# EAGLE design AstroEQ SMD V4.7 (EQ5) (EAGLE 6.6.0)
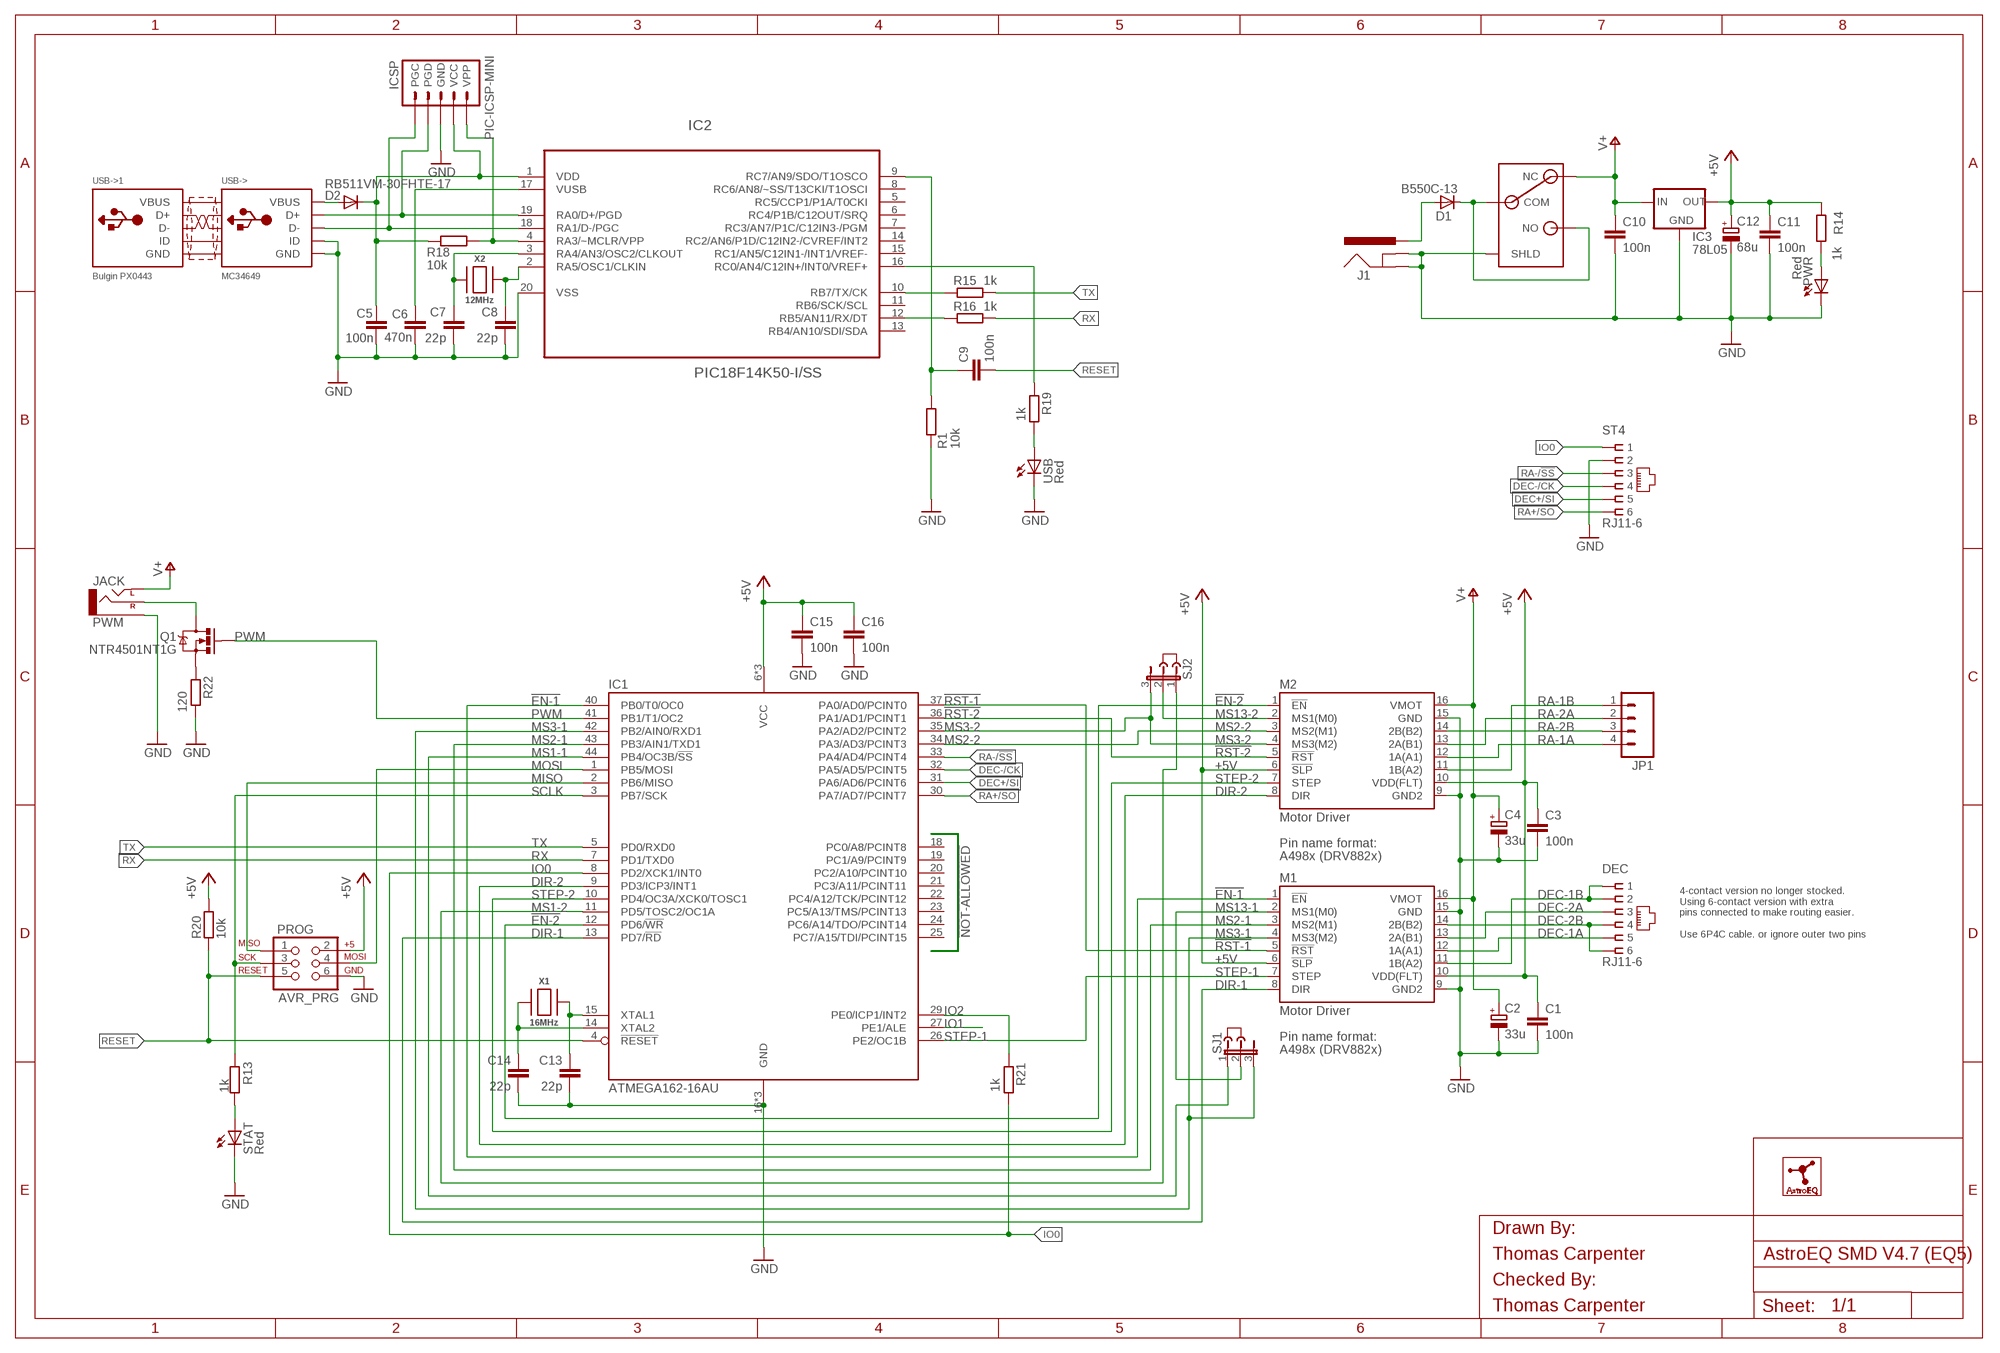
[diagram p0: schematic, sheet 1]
FRAME1 (A3L-LOC): CHECKED_BY: Thomas Carpenter; DRAWN_BY: Thomas Carpenter
USB->1 (USB-PANEL): MF: BULGIN; MPN: PX0443; OC_FARNELL: 1229685

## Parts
C1  100n  C-EUC0603  [C0603]
C2  33u  CPOL-EUSMCC  [SMC_C]
C3  100n  C-EUC0603  [C0603]
C4  33u  CPOL-EUSMCC  [SMC_C]
C5  100n  C-EUC0603  [C0603]
C6  470n  C-EUC0603  [C0603]
C7  22p  C-EUC0603  [C0603]
C8  22p  C-EUC0603  [C0603]
C9  100n  C-EUC0603  [C0603]
C10  100n  C-EUC0603  [C0603]
C11  100n  C-EUC0603  [C0603]
C12  68u  CPOL-EUSMCC  [SMC_C]
C13  22p  C-EUC0603  [C0603]
C14  22p  C-EUC0603  [C0603]
C15  100n  C-EUC0603  [C0603]
C16  100n  C-EUC0603  [C0603]
D1  B550C-13  DIODE-SMC  [SMC]
D2  RB511VM-30FHTE-17  DIODESOD  [SOD-323]
DEC  RJ11-6  RJ11-2L-B  [RJ11-NO_SHIELD]
IC1  ATMEGA162-16AU  [TQFP44]
IC2  PIC18F14K50-I/SS  [SS20]
IC3  78L05  78LXXSOT-23  [SOT23]
ICSP  PIC-ICSP-MINI  [PIC-ICSP-MINI]
J1  POWER_JACKPANEL  [POWER_JACK_PANEL]
J2  JUMPER  [JUMP]
J3  JUMPER  [JUMP]
JP1  M04POLAR  [MOLEX-1X4]
LOGO1  ASTROEQ5MM  [ASTROEQ-SMALL]
M1  Motor Driver  A4983CARRIER  [DIP16-W]
M2  Motor Driver  A4983CARRIER  [DIP16-W]
PROG  AVR_PRG  AVR_SPI_PRG_6PTH  [2X3]
PWM  JACK  AUDIO-JACKVERT  [AUDIO-JACK-3.5MM-VERT]
PWR  Red  LED3MM  [LED3MM]
PWR-SW  SWITCH  [SPST]
Q1  NTR4501NT1G  MOSFET-NCHANNELSMD  [SOT23-3]
R1  10k  R-EU_R0603  [R0603]
R13  1k  R-EU_R0603  [R0603]
R14  1k  R-EU_R0603  [R0603]
R15  1k  R-EU_R0603  [R0603]
R16  1k  R-EU_R0603  [R0603]
R18  10k  R-EU_R0603  [R0603]
R19  1k  R-EU_R0603  [R0603]
R20  10k  R-EU_R0603  [R0603]
R21  1k  R-EU_R0603  [R0603]
R22  120  R-EU_R0805  [R0805]
SJ1  JP2E  [JP2]
SJ2  JP2E  [JP2]
ST4  RJ11-6  RJ11-2L-B  [RJ11-NO_SHIELD]
STAT  Red  LED3MM  [LED3MM]
USB  Red  LED3MM  [LED3MM]
USB->  MC34649  USBBULGINWIRE  [22-23-2051]
X1  16MHz  XTALNX5032  [NX5032]
X2  12MHz  XTALNX5032  [NX5032]

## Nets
!EN-1: IC1.40(PB0/T0/OC0) M1.1(!EN)
!EN-2: IC1.12(PD6/!WR) M2.1(!EN)
!RST-1: IC1.37(PA0/AD0/PCINT0) M1.5(!RST)
!RST-2: IC1.36(PA1/AD1/PCINT1) M2.5(!RST)
+5V: C1.1 C3.1 C11.1 C12.+ C15.1 C16.1 IC1.6(VCC) IC1.17(VCC) IC1.38(VCC) IC3.1(OUT) M1.6(!SLP) M1.10(VDD(FLT)) M2.6(!SLP) M2.10(VDD(FLT)) PROG.2 R14.1 R20.2
AVROSC1: C13.1 IC1.15(XTAL1) X1.P$1
AVROSC2: C14.1 IC1.14(XTAL2) X1.P$2
D_N [usbdat]: IC2.18(RA1/D-/PGC) ICSP.5(PGC) USB->.2(D-)
D_P [usbdat]: IC2.19(RA0/D+/PGD) ICSP.4(PGD) USB->.3(D+)
DEC+/SI: IC1.31(PA6/AD6/PCINT6) ST4.5
DEC-1A: DEC.5 M1.12(1A(A1))
DEC-1B: DEC.1 DEC.2 M1.11(1B(A2))
DEC-2A: DEC.3 M1.13(2A(B1))
DEC-2B: DEC.4 DEC.6 M1.14(2B(B2))
DEC-/CK: IC1.32(PA5/AD5/PCINT5) ST4.4
DIR-1: IC1.13(PD7/!RD) M1.8(DIR)
DIR-2: IC1.9(PD3/ICP3/INT1) M2.8(DIR)
DTR: C9.1 IC2.9(RC7/AN9/SDO/T1OSCO) R1.1
GND: C1.2 C2.- C3.2 C4.- C5.2 C6.1 C7.2 C8.2 C10.2 C11.2 C12.- C13.2 C14.2 C15.2 C16.2 IC1.16(GND) IC1.28(GND) IC1.39(GND) IC2.20(VSS) IC3.3(GND) ICSP.3(GND) J1.SHUNT(GNDBREAK) J1.SLEEVE(GND) M1.9(GND2) M1.15(GND) M2.9(GND2) M2.15(GND) PROG.6 PWM.1(SLEEVE) PWR-SW.S1(SHLD) PWR-SW.S2(SHLD) PWR-SW.S3(SHLD) PWR-SW.S4(SHLD) PWR.K(C) R1.2 R22.1 ST4.2 STAT.K(C) USB->.4(GND) USB->.5(ID) USB.K(C)
IO0: IC1.8(PD2/XCK1/INT0) R21.1 ST4.1
IO1: IC1.27(PE1/ALE)
IO2: IC1.29(PE0/ICP1/INT2) R21.2
MCLR: IC2.4(RA3/~MCLR/VPP) ICSP.1(VPP) R18.1
MISO: IC1.2(PB6/MISO) PROG.1
MOSI: IC1.1(PB5/MOSI) PROG.4
MS1-1: IC1.44(PB4/OC3B/!SS) SJ1.1
MS1-2: IC1.11(PD5/TOSC2/OC1A) SJ2.1
MS2-1: IC1.43(PB3/AIN1/TXD1) M1.3(MS2(M1))
MS2-2: IC1.34(PA3/AD3/PCINT3) M2.3(MS2(M1))
MS3-1: IC1.42(PB2/AIN0/RXD1) M1.4(MS3(M2)) SJ1.3
MS3-2: IC1.35(PA2/AD2/PCINT2) M2.4(MS3(M2)) SJ2.3
MS13-1: M1.2(MS1(M0)) SJ1.2
MS13-2: M2.2(MS1(M0)) SJ2.2
PWM: IC1.41(PB1/T1/OC2) Q1.1(G)
PWM-OUT: PWM.3(RIGHT) Q1.3(D)
PWM-RES: Q1.2(S) R22.2
PWRLED: PWR.A R14.2
RA+/SO: IC1.30(PA7/AD7/PCINT7) ST4.6
RA-1A: JP1.4 M2.12(1A(A1))
RA-1B: JP1.1 M2.11(1B(A2))
RA-2A: JP1.2 M2.13(2A(B1))
RA-2B: JP1.3 M2.14(2B(B2))
RA-/!SS: IC1.33(PA4/AD4/PCINT4) ST4.3
RESET: C9.2 IC1.4(!RESET) PROG.5 R20.1
RX: IC1.7(PD1/TXD0) R16.1
RX(USB): IC2.12(RB5/AN11/RX/DT) R16.2
SCLK: IC1.3(PB7/SCK) PROG.3 R13.1
STATLED: R13.2 STAT.A
STEP-1: IC1.26(PE2/OC1B) M1.7(STEP)
STEP-2: IC1.10(PD4/OC3A/XCK0/TOSC1) M2.7(STEP)
SWITCH: D1.C PWR-SW.COM PWR-SW.NO
TX: IC1.5(PD0/RXD0) R15.1
TX(USB): IC2.10(RB7/TX/CK) R15.2
USBLED: R19.1 USB.A
USBOSC1: C8.1 IC2.2(RA5/OSC1/CLKIN) X2.P$2
USBOSC2: C7.1 IC2.3(RA4/AN3/OSC2/CLKOUT) X2.P$1
USBSTAT: IC2.16(RC0/AN4/C12IN+/INT0/VREF+) R19.2
V+: C2.+ C4.+ C10.1 IC3.2(IN) M1.16(VMOT) M2.16(VMOT) PWM.2(LEFT) PWR-SW.NC
VBUS: D2.2(A) USB->.1(VBUS)
VIN: D1.A J1.CENTRE(PWR)
VPIC: C5.1 D2.1(C) IC2.1(VDD) ICSP.2(VCC) R18.2
VUSB: C6.2 IC2.17(VUSB)
Unconnected: IC1.18(PC0/A8/PCINT8) IC1.19(PC1/A9/PCINT9) IC1.20(PC2/A10/PCINT10) IC1.21(PC3/A11/PCINT11) IC1.22(PC4/A12/TCK/PCINT12) IC1.23(PC5/A13/TMS/PCINT13) IC1.24(PC6/A14/TDO/PCINT14) IC1.25(PC7/A15/TDI/PCINT15) IC2.5(RC5/CCP1/P1A/T0CKI) IC2.6(RC4/P1B/C12OUT/SRQ) IC2.7(RC3/AN7/P1C/C12IN3-/PGM) IC2.8(RC6/AN8/~SS/T13CKI/T1OSCI) IC2.11(RB6/SCK/SCL) IC2.13(RB4/AN10/SDI/SDA) IC2.14(RC2/AN6/P1D/C12IN2-/CVREF/INT2) IC2.15(RC1/AN5/C12IN1-/INT1/VREF-)

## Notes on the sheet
- 4-contact version no longer stocked.
  Using 6-contact version with extra
  pins connected to make routing easier.
  
  Use 6P4C cable. or ignore outer two pins

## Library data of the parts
C1 C3 C5 C9-C11 C15 C16 = rcl:C-EU: CAPACITOR, European symbol; MF: MULTICOMP; MPN: MC0603F104Z250CT; OC_FARNELL: 1759038
C2 C4 = rcl:CPOL-EU: POLARIZED CAPACITOR, European symbol; MF: KEMET; MPN: T491C336K025AT; OC_FARNELL: 1793896
C6 = rcl:C-EU: CAPACITOR, European symbol; MF: MULTICOMP; MPN: MC0603F474Z160CT; OC_FARNELL: 1759021
C7 C8 C13 C14 = rcl:C-EU: CAPACITOR, European symbol; MF: MULTICOMP; MPN: MC0603N220J500CT; OC_FARNELL: 1759057
C12 = rcl:CPOL-EU: POLARIZED CAPACITOR, European symbol; MF: AVX; MPN: TPSC686K016R0125; OC_FARNELL: 1658976
D1 = diode:DIODE-: DIODE; MF: DIODES INC.; MPN: B550C-13-F; OC_FARNELL: 1858608
D2 = SparkFun:DIODE: Diode; MF: ROHM; MPN: RB511VM-30FHTE-17; OC_FARNELL: 2581544
DEC ST4 = con-tycoelectronics:RJ11: CORCOM Modular RJ Jacks No Shield Source: www.tycoelectronics.com .. ENG_DS_1654001_1099_RJ_L_0507.pdf; MF: MOLEX; MPN: 95503-2661; OC_FARNELL: 1620210
IC1 = atmel:ATMEGA162: 8-bit RISC MICROCONTROLLER 16K Bytes internal flash program memory 1K Bytes internal SRAM Upto 64K Bytes optional external memory space 512 Bytes EEPROM Two 8-bit timers Two 16-bit timers Dual programmable serial USARTs Master/Slave serial SPI interface Source: ATMEGA162_DIP40.lbr; MF: ATMEL; MPN: ATMEGA162-16AU; OC_FARNELL: 9171150
IC2 = microchip:PIC18F14K50: USB Flash Microcontrollers; MF: MICROCHIP
IC3 = v-reg:78LXX: VOLTAGE REGULATOR; MF: TAIWAN SEMICONDUCTOR; MPN: TS78L05CX RFG; OC_FARNELL: 1476698
ICSP = SparkFun:PIC-ICSP-MINI: PIC-ICSP-Mini Miniature 5-pin connection for temporary programming of PICs. Use this device in your design to save space. Program the PIC with this adapter Spark Fun Electronics SKU : BOB-00194; OC_FARNELL: unknown
J1 = SparkFun:POWER_JACK: Power Jack This is the standard 5.5mm barrel jack for power. The PTH is the most common, proven, reliable, footprint. All others are experimental. The Slot footprint only works if the mill layer is transmitted to the PCB fab house so be warned. Spark Fun Electronics SKU : PRT-00119. Mating wall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; MF: SWITCHCRAFT; MPN: PCL712AS; OC_FARNELL: 1871167
J2 J3 = jumper:JUMPER: JUMPER header; MF: 3M; MPN: 969102-0000-DA; OC_FARNELL: 2579814
JP1 = SparkFun:M04: Header 4 Standard 4-pin 0.1" header. Use with straight break away headers (SKU : PRT-00116), right angle break away headers (PRT-00553), swiss pins (PRT-00743), machine pins (PRT-00117), and female headers (PRT-00115). Molex polarized connector foot print use with SKU : PRT-08231 with associated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; MF: MULTICOMP; MPN: MC34645; OC_FARNELL: 1675775
LOGO1 = AstroEQTooth:ASTROEQ; OC_FARNELL: unknown
M1 M2 = A4983Carrier:A4983CARRIER; MF: SAMTEC; MPN: CES-116-01-T-S; OC_FARNELL: 1667522
PROG = SparkFun:AVR_SPI_PRG_6: AVR ISP 6 Pin This is the reduced ISP connector for AVR programming. Common on Arduino. This footprint will take up less PCB space and can be used with a 10-pin to 6-pin adapter such as SKU: BOB-08508; MF: AMP - TE CONNECTIVITY; MPN: 826632-3; OC_FARNELL: 3418492
PWM = SparkFun:AUDIO-JACK: 3.5mm Audio Jack Simple 3.5mm common PCB mount audio jack. SKU: PRT-08032; MANUFACTURER: LUMBERG; MF: LUMBERG; MPN: 1502 01; OC_FARNELL: 1243242
PWR STAT USB = led:LED: LED; MF: KINGBRIGHT; MPN: L-424HDT; OC_FARNELL: 1142499
PWR-SW = con-tycoelectronics:SWITCH; MF: TE CONNECTIVITY; MPN: AE101J1V3B004; OC_FARNELL: 1813654
Q1 = SparkFun:MOSFET-NCHANNEL; MF: ON SEMICONDUCTOR; MPN: NTR4501NT1G; OC_FARNELL: 1431305
R1 R18 R20 = rcl:R-EU_: RESISTOR, European symbol; MF: MULTICOMP; MPN: MCWR06X1002FTL; OC_FARNELL: 2447230
R13-R16 R19 R21 = rcl:R-EU_: RESISTOR, European symbol; MF: MULTICOMP; MPN: MCWR06X1001FTL; OC_FARNELL: 2447272
R22 = rcl:R-EU_: RESISTOR, European symbol; MF: MULTICOMP; MPN: MCWR08X1200FTL; OC_FARNELL: 2447561
SJ1 SJ2 = jumper:JP2E: JUMPER; MF: MULTICOMP; MPN: 2211S-03G; OC_FARNELL: 1593412
USB-> = adafruit:USB: USB Connectors USBMINIB - Surface Mount Female Mini-B USB Connector 4UConnector: 06564 By microbuilder.eu Thru-hole RA Female Mini-B USB Connector 4UConnector: 18732 By ladyada.net; MF: MULTICOMP; MPN: MC34649; OC_FARNELL: 1675777
X1 = adafruit:XTAL: Low cost SMT crystals, no capacitors included; MF: TXC; MPN: 7A-16.000MAAJ-T; OC_FARNELL: 1841946
X2 = adafruit:XTAL: Low cost SMT crystals, no capacitors included; MF: TXC; MPN: 7A-12.000MAAJ-T; OC_FARNELL: 1841940

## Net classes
1 power: width 0.61 mm, drill 0.711 mm, clearance 0.203 mm
2 gnd: width 0.305 mm, drill 0.711 mm, clearance 0.203 mm
3 usbvcc: width 0.508 mm, drill 0.711 mm, clearance 0.203 mm
4 usbdat: width 0.406 mm, clearance 0.152 mm

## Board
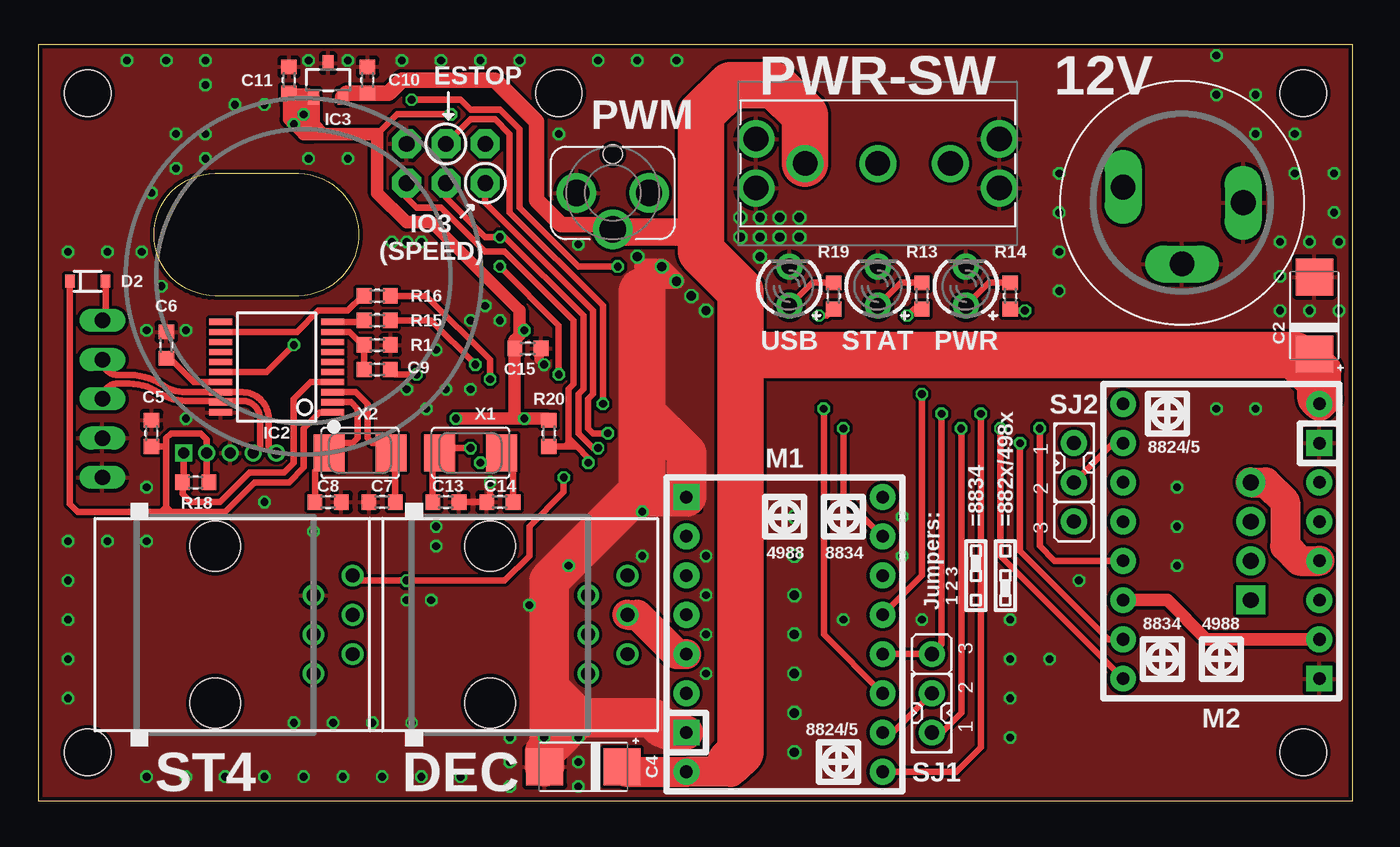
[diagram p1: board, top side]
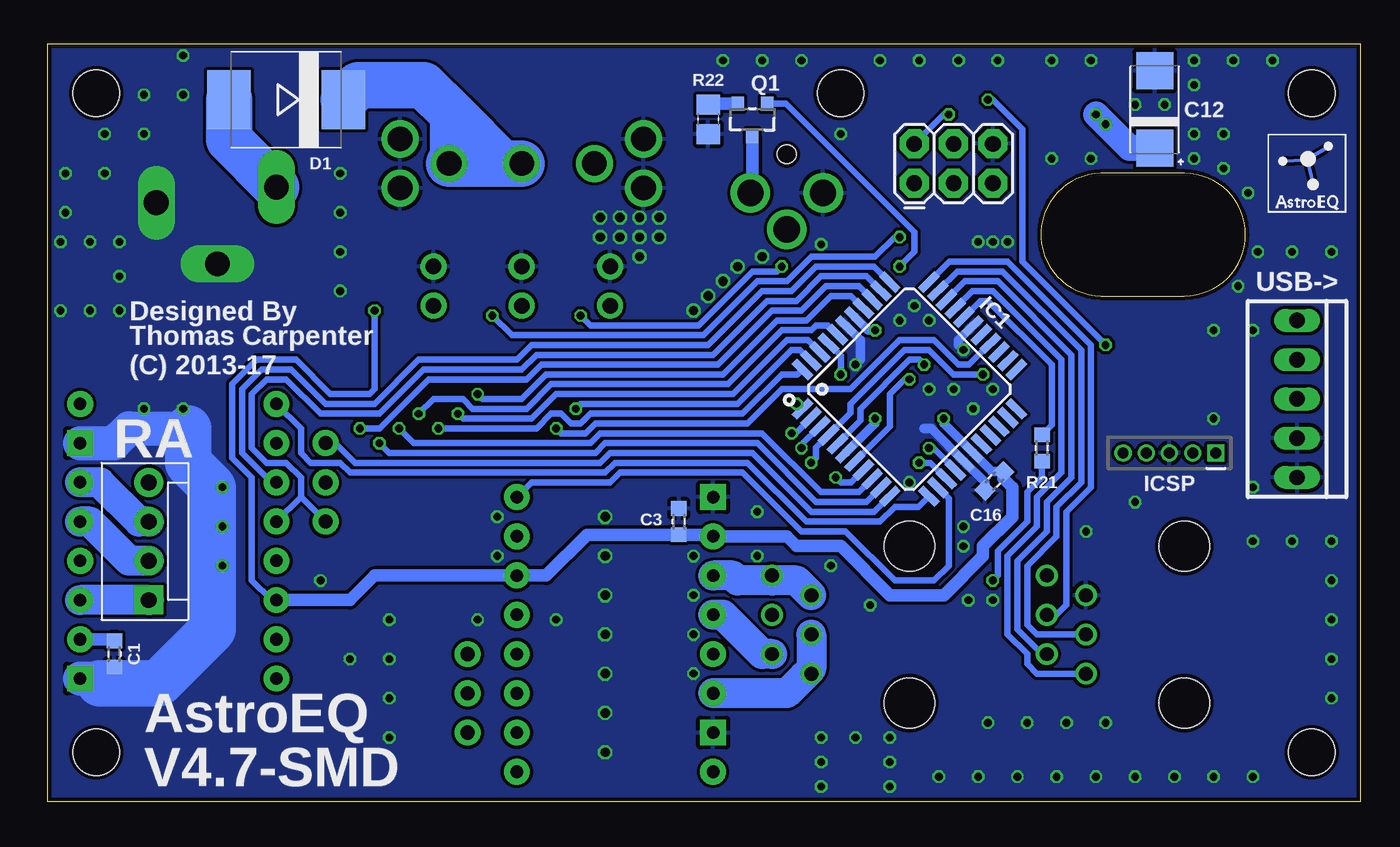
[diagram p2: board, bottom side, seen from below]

Size 85 x 49 mm. Coordinates in mm from the lower left corner, seen from the top.
Outline: 0,0 0,49 85,49 85,0 0,0
Outline: 16.83,40.64 arc-177 16.83,32.7 11.43,32.7 arc-180 11.43,40.64 16.83,40.64
Copper layers (1*16): Top 0.035mm / dielectric 1.5mm / Bottom 0.035mm
Design rules "ITEADstudio_DRC *": minimum track width 6mil, minimum drill 12mil, track to track 6mil, track to pad 6mil, pad to pad 6mil, via to via 6mil, smd to smd 0mil, copper to edge 10mil, drill to drill 10mil, minimum pad ring 8mil, minimum via ring 6mil, stop-mask expansion 2mil, vias tented up to drill 1mm, thermal gap 10mil
Holes 3 mm at 81.83,3.17 33.66,45.83 3.17,45.83 81.83,45.83 3.17,3.17

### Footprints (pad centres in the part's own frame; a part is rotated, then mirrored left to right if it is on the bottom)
C0603 = smd 0.95 x 1: 1 -0.85,0; 2 0.85,0
SMC_C = smd 2.4 x 2.4: + -2.5,0; - 2.5,0
SMC = smd 2.8 x 3.8: A 3.7,0; C -3.7,0
SOD-323 = smd 0.63 x 0.83: 1 -1.15,0; 2 1.15,0
RJ11-NO_SHIELD = drill 0.9 pad 1.4: 1 -3.175,8.89; 2 -1.905,6.35; 3 -0.635,8.89; 4 0.635,6.35; 5 1.905,8.89; 6 3.175,6.35 | hole 3.251: -5.08,0; 5.08,0
TQFP44 = smd 1.5 x 0.5: 1 -5.8,4; 2 -5.8,3.2; 3 -5.8,2.4; 4 -5.8,1.6; 5 -5.8,0.8; 6 -5.8,0; 7 -5.8,-0.8; 8 -5.8,-1.6; 9 -5.8,-2.4; 10 -5.8,-3.2; 11 -5.8,-4; 23 5.8,-4; 24 5.8,-3.2; 25 5.8,-2.4; 26 5.8,-1.6; 27 5.8,-0.8; 28 5.8,0; 29 5.8,0.8; 30 5.8,1.6; 31 5.8,2.4; 32 5.8,3.2; 33 5.8,4 | smd 0.5 x 1.5: 12 -4,-5.8; 13 -3.2,-5.8; 14 -2.4,-5.8; 15 -1.6,-5.8; 16 -0.8,-5.8; 17 0,-5.8; 18 0.8,-5.8; 19 1.6,-5.8; 20 2.4,-5.8; 21 3.2,-5.8; 22 4,-5.8; 34 4,5.8; 35 3.2,5.8; 36 2.4,5.8; 37 1.6,5.8; 38 0.8,5.8; 39 0,5.8; 40 -0.8,5.8; 41 -1.6,5.8; 42 -2.4,5.8; 43 -3.2,5.8; 44 -4,5.8
SS20 = smd 0.4 x 1.5: 1 -2.925,-3.625; 2 -2.275,-3.625; 3 -1.625,-3.625; 4 -0.975,-3.625; 5 -0.325,-3.625; 6 0.325,-3.625; 7 0.975,-3.625; 8 1.625,-3.625; 9 2.275,-3.625; 10 2.925,-3.625; 11 2.925,3.625; 12 2.275,3.625; 13 1.625,3.625; 14 0.975,3.625; 15 0.325,3.625; 16 -0.325,3.625; 17 -0.975,3.625; 18 -1.625,3.625; 19 -2.275,3.625; 20 -2.925,3.625
SOT23 = smd 0.7 x 1: 1 -0.95,-1.1; 2 0.95,-1.1; 3 0,1.1
PIC-ICSP-MINI = drill 0.7 square: 1 -3,0 | drill 0.7: 2 -1.5,0; 3 0,0; 4 1.5,0; 5 3,0
POWER_JACK_PANEL = drill 1.6 long: CENTRE 3.81,-1.016; SHUNT -3.962,0; SLEEVE 0,3.962
MOLEX-1X4 = drill 1.016 pad 1.88 square: 1 0,0 | drill 1.016 pad 1.88: 2 2.54,0; 3 5.08,0; 4 7.62,0
DIP16-W = drill 0.813 pad 1.676: 1 -8.89,-6.35; 2 -6.35,-6.35; 3 -3.81,-6.35; 4 -1.27,-6.35; 5 1.27,-6.35; 6 3.81,-6.35; 7 6.35,-6.35; 8 8.89,-6.35; 10 6.35,6.35; 11 3.81,6.35; 12 1.27,6.35; 13 -1.27,6.35; 14 -3.81,6.35; 16 -8.89,6.35 | drill 0.813 pad 1.676 square: 9 8.89,6.35; 15 -6.35,6.35
2X3 = drill 1.016 pad 1.88 octagon: 1 -2.54,-1.27; 2 -2.54,1.27; 3 0,-1.27; 4 0,1.27; 5 2.54,-1.27; 6 2.54,1.27
AUDIO-JACK-3.5MM-VERT = drill 1.7: 1 2.35,0; 2 0,2.35; 3 -2.35,0 | hole 1.2: 0,-2.5
LED3MM = drill 1 pad 1.676: A -1.27,0; K 1.27,0
SPST = drill 1.6: COM 0,0; NC -4.699,0; NO 4.699,0; S1 7.874,1.587; S2 7.874,-1.587; S3 -7.874,1.587; S4 -7.874,-1.587
SOT23-3 = smd 0.8 x 0.9: 1 -0.95,-1; 2 0.95,-1; 3 0,1.1
R0603 = smd 0.95 x 1: 1 -0.85,0; 2 0.85,0
R0805 = smd 1.3 x 1.5: 1 -0.95,0; 2 0.95,0
JP2 = drill 0.914 pad 1.676: 1 -2.54,0; 2 0,0; 3 2.54,0
22-23-2051 = drill 1 long: 1 -5.08,0; 2 -2.54,0; 3 0,0; 4 2.54,0; 5 5.08,0
NX5032 = smd 2 x 2.4: P$1 2,0; P$2 -2,0

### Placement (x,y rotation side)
C1  80.64,9.53 270 bottom
C2  82.55,31.43 90 top
C3  44.13,18.1 90 bottom
C4  35.24,2.22 180 top
C5  7.3,23.81 90 top
C6  8.26,29.53 270 top
C7  22.23,19.37 180 top
C8  18.73,19.37 0 top
C9  21.91,27.94 0 top
C10  21.27,46.67 90 top
C11  16.19,46.67 90 top
C12  13.34,44.77 90 bottom
C13  26.35,19.37 0 top
C14  29.84,19.37 180 top
C15  31.66,29.3 0 top
C16  23.72,20.73 225 bottom
D1  69.53,45.4 180 bottom
D2  3.17,33.66 0 top
DEC  29.21,11.43 270 top
IC1  29.21,26.67 45 bottom
IC2  15.4,28.1 90 top
IC3  18.73,46.67 0 top
ICSP  12.38,22.54 180 bottom
J1  73.98,38.73 180 top
J2  57.78,5.71 0 top
J3  66.99,21.91 0 top
JP1  78.42,13.02 90 bottom
LOGO1  6.03,38.1 0 bottom
M1  48.26,10.79 90 top
M2  76.52,16.83 270 top
PROG  26.35,41.27 0 bottom
PWM  37.15,39.37 180 top
PWR  60.01,33.34 90 top
PWR-SW  54.29,41.27 0 top
Q1  39.37,44.13 180 bottom
R1  21.91,29.53 0 top
R13  57.15,32.7 90 top
R14  62.87,32.7 90 top
R15  21.91,31.11 180 top
R16  21.91,32.7 180 top
R18  10.16,20.64 0 top
R19  51.44,32.7 270 top
R20  33.02,23.81 90 top
R21  20.64,22.86 90 bottom
R22  42.23,44.13 90 bottom
SJ1  57.78,6.99 90 top
SJ2  66.99,20.64 270 top
ST4  11.43,11.43 270 top
STAT  54.29,33.34 90 top
USB  48.58,33.34 90 top
USB->  4.13,26.04 270 bottom
X1  27.94,22.54 180 top
X2  20.8,22.54 0 top

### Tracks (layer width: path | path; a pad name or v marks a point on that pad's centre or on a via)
!EN-1  (via drill 0.5)
  Top 0.406: M1.1 59.37,1.91 60.96,3.49 v60.96,25.08
  Bottom 0.406: IC1.40 34.47,30.8 35.24,30.8 35.56,30.48 37.47,30.48 40.96,26.99 52.39,26.99 53.98,25.4 57.47,25.4 58.1,26.04 60.01,26.04 v60.96,25.08
!EN-2
  Bottom 0.406: IC1.12 28.63,19.05 30.16,19.05 31.11,18.1 35.88,18.1 39.69,21.91 48.26,21.91 48.9,21.27 65.41,21.27 66.04,21.91 67.94,21.91 68.58,22.54 68.58,24.13 M2.1
!RST-1  (via drill 0.5)
  Top 0.406: M1.5 57.15,14.61 v57.15,26.35
  Bottom 0.406: IC1.37 32.98,32.7 34.29,32.7 35.88,31.11 37.78,31.11 41.27,27.62 52.7,27.62 54.29,26.04 56.83,26.04 v57.15,26.35
!RST-2  (via drill 0.5)
  Top 0.406: M2.5 65.72,15.56 64.77,16.51 v64.77,24.13
  Bottom 0.406: IC1.36 32.48,33.34 34.61,33.34 36.2,31.75 38.1,31.75 41.59,28.26 53.02,28.26 53.98,27.3 60.33,27.3 63.5,24.13 v64.77,24.13
+5V  (via drill 0.5)
  Top 0.406: 31.11,30.16 30.8,29.84 | v26.67,44.45 23.18,44.45 21.91,43.18 | R14.1 62.97,31.75 v63.82,31.75
  Top 0.813: R20.2 32.92,24.77 v31.43,24.77 30.8,24.77 | v26.99,24.77 30.8,24.77 | 30.8,24.77 30.8,29.29 C15.1 30.81,29.86 v31.43,30.48 31.11,30.8 | 31.11,30.8 31.11,31.75 25.4,37.47 23.81,37.47 21.91,39.37 21.91,43.18 18.41,43.18 | 31.11,30.8 31.11,30.16 | M2.6 73.03,13.02 75.56,10.48 M2.10 | 18.41,43.18 17.78,43.81 | 17.78,43.81 IC3.1 | 16.19,45.4 C11.1 16.41,45.82 16.51,45.72 | 16.19,45.4 16.83,44.77 16.83,44.45 16.19,45.09 | 16.19,45.09 16.19,45.4 | 16.19,45.09 16.19,44.13 v16.51,43.81 17.14,43.18 17.78,43.18 | 18.41,43.18 17.78,43.18 | 17.78,43.18 17.14,43.81 v17.14,44.45 17.78,43.81 | 16.51,45.72 17.78,44.45 17.78,45.4 17.46,45.72 16.51,45.72
  Bottom 0.406: PROG.2 26.99,44.45 v26.67,44.45 | v63.82,31.75 63.82,26.67 64.14,26.35 66.67,26.35 68.9,28.57 71.44,28.57 73.03,26.99 73.03,22.23 71.75,20.95 71.75,14.29 70.48,13.02 M2.6
  Bottom 0.61: C16.1 23.87,21.33 IC1.17 26.99,24.45 v26.99,24.77 | v31.43,24.77 31.43,24.45 IC1.6 | IC1.38 31.89,30.48 v31.43,30.48
  Bottom 0.813: C16.1 23.12,20.9 22.54,20.32 22.54,18.41 24.45,16.51 24.45,15.88 26.99,13.34 30.48,13.34 33.66,16.51 36.51,16.51 37.15,17.14 M1.10 42.01,17.25 C3.1 50.06,17.25 52.7,14.61 M1.6 63.82,14.61 65.41,13.02 M2.6 | 80.54,10.48 C1.1 80.75,10.48 M2.10
  Bottom 1.676: C12.+ 14.96,42.27 v17.14,44.45
AVROSC1  (via drill 0.5)
  Top 0.406: v27.94,22.86 26.26,22.86 X1.P$1 25.5,22.11 C13.1
  Bottom 0.406: IC1.15 27.66,22.86 v27.94,22.86
AVROSC2  (via drill 0.5)
  Top 0.406: v28.57,21.91 29.3,21.91 X1.P$2 30.7,21.79 C14.1
  Bottom 0.406: IC1.14 27.84,21.91 v28.57,21.91
D_N
  Top 0.406: USB->.2 arc90 5.12,27.58 5.87,27.58 arc-34 8.1,26.9 arc35 9.52,26.47 IC2.18 | ICSP.5 arc-90 14.88,23.04 14.88,24.77 arc90 13.18,26.47 IC2.18 | IC2.18
D_P
  Top 0.406: USB->.3 arc-90 5.12,27.03 5.87,27.03 arc-34 7.78,26.44 arc35 9.53,25.91 11.77,25.91 | ICSP.4 arc90 14.33,22.99 14.33,24.77 arc90 13.18,25.91 11.77,25.91 | IC2.19 11.77,25.91
DEC+/SI
  Bottom 0.406: IC1.31 25.62,33.66 23.5,33.66 18.73,28.89 18.73,20.95 20.32,19.37 20.32,17.46 22.23,15.56 22.23,11.11 20.64,9.53 ST4.5
DEC-1A
  Bottom 1.93: DEC.5 38.73,9.53 41.27,12.06 M1.12
DEC-1B
  Bottom 0.406: DEC.1 38.1,14.29
  Bottom 1.93: DEC.2 36.51,14.29 38.1,14.29 40.32,14.29 40.64,14.61 M1.11
DEC-2A
  Top 1.93: DEC.3 38.73,12.06 41.27,9.53 M1.13
DEC-2B
  Bottom 0.406: DEC.6 36.04,8.26 36.04,8.1
  Bottom 1.93: DEC.4 35.56,8.57 36.04,8.1 37.15,6.99 M1.14
DEC-/CK
  Bottom 0.406: IC1.32 26.11,34.29 23.18,34.29 18.1,29.21 18.1,20.64 19.68,19.05 19.68,17.14 21.59,15.24 21.59,11.43 20.95,10.79 ST4.4
DIR-1
  Bottom 0.406: IC1.13 26.67,19.61 26.67,15.24 27.62,14.29 30.16,14.29 33.34,17.46 36.2,17.46 40.01,21.27 47.94,21.27 48.58,20.64 53.66,20.64 M1.8
DIR-2  (via drill 0.5)
  Top 0.406: M2.8 62.23,15.88 v62.23,24.13
  Bottom 0.406: IC1.9 32.48,20 34.92,20 38.73,23.81 49.21,23.81 49.85,23.18 61.28,23.18 v62.23,24.13
DTR
  Top 0.406: IC2.9 20.11,30.37 20.95,29.53 R1.1 C9.1
GND  (via drill 0.5, 0.6)
  Top 0.406: C13.2 C14.2 29.21,19.58 v29.21,20.64
  Top 0.61: C15.2 32.38,29.18 32.38,28.57 v32.7,28.26
  Top 1.016: 39.05,34.61 v40.32,34.61 v41.27,33.66 38.42,33.66 38.42,33.02 39.05,33.02
  Top 2.184: 40.32,4.76 40.64,4.45 M1.15
  Top 2.54: C4.- 32.74,3.21 33.02,3.49 | 33.02,3.49 34.92,5.4 | 34.92,5.4 39.69,5.4 40.32,4.76 | 34.92,5.4 33.02,7.3 | 33.02,7.3 33.02,14.29 38.42,19.68 M1.9 41.91,22.54 39.05,25.4 | 33.02,7.3 33.02,3.49
  Top 3: 39.05,20.32 39.05,25.4 39.05,33.02
  Bottom 0.61: C16.2 24.32,20.65 IC1.16 27.8,24.13 28.26,24.13 | IC1.28 26.04,29.84 26.04,29.53 v25.72,29.21 | IC1.39 32.38,29.84 32.38,28.57 v32.7,28.26
  Bottom 0.813: C1.2 81.38,7.94
  Bottom 2.184: 81.38,7.94 M2.9 | M2.15 80.64,23.18 79.69,24.13 75.88,24.13
  Bottom 3: 75.88,24.13 75.88,21.91 74.3,20.32 74.3,11.11 77.79,7.62 81.6,7.62
  other vias: 14.61,19.37 17.78,17.46 25.72,17.78 9.53,24.77 9.53,30.48 25.72,16.51 47.94,36.51 43.18,31.75 46.67,35.24 23.81,26.67 27.94,26.67 27.94,31.11 29.84,31.11 25.08,25.4 26.35,26.67 45.4,36.51 46.67,36.51 22.86,36.2 28.89,32.07 49.21,36.51 47.94,37.78 49.21,37.78 45.4,37.78 46.67,37.78 42.23,32.7 48.9,3.17 48.9,5.71 48.9,8.26 48.9,10.79 48.9,13.34 48.9,15.88 48.9,18.41 23.81,13.02 25.4,13.02 34.29,15.24 39.05,18.73 30.48,0.95 30.48,4.13 34.92,4.13 34.92,0.95 32.7,4.13 30.48,2.54 34.92,2.54 43.18,8.26 43.18,10.79 43.18,13.34 43.18,15.88 39.05,15.88 38.73,35.24 23.81,36.2 24.77,36.2 34.92,36.04 84.14,36.2 84.14,31.75 82.23,36.2 80.33,36.2 80.33,33.97 80.33,31.75 82.23,31.75 10.79,47.94 10.79,46.35 12.7,45.09 14.61,45.09 17.46,47.94 20,47.94 23.5,47.94 26.04,47.94 28.57,47.94 31.11,47.94 36.2,47.94 38.73,47.94 41.27,47.94 33.66,43.18 7.94,33.34 8.89,40.96 8.89,43.18 10.79,43.18 20,41.59 1.91,16.83 1.91,14.29 1.91,11.75 1.91,9.21 1.91,6.67 22.23,1.59 19.68,1.59 17.14,1.59 14.61,1.59 12.06,1.59 9.53,1.59 6.99,1.59 24.77,1.59 27.3,1.59 62.87,9.21 65.41,9.21 62.87,6.67 62.87,4.13 73.66,15.24 73.66,17.78 73.66,20.32 76.2,25.4 78.74,25.4 66.04,33.02 66.04,35.56 78.74,45.72 81.28,43.18 83.82,40.64 81.28,40.64 78.74,43.18 76.2,48.26 76.2,45.72 83.82,38.1 6.99,30.48 6.99,20.32 4.45,16.83 6.99,16.83 1.91,35.56 4.45,35.56 6.67,35.56 17.46,41.59 10.79,41.59 7.3,39.37 8.26,47.94 5.71,47.94 31.75,12.7 16.51,5.08 19.05,5.08 21.59,5.08 24.13,5.08 62.87,11.75 57.15,11.75 67.31,14.29 52.07,11.75 55.88,18.41 55.88,15.88 66.04,38.1 66.04,40.64
  pour Bottom (isolate 0.203): -2.54,50.8 86.36,50.8 86.36,-2.54 -2.54,-2.54
  pour Top (isolate 0.203): -2.54,50.8 86.36,50.8 86.36,-2.54 -2.54,-2.54
  pour Bottom (isolate 0.203, no thermals): 78.74,43.18 76.2,43.18 71.12,38.1 71.12,33.02 81.28,33.02 81.28,40.64
IO0  (via drill 0.5)
  Top 0.406: ST4.1 20.64,14.29 v23.81,14.29 30.16,14.29 31.75,15.88 31.75,17.78 33.97,20 v33.97,20.95
  Bottom 0.406: R21.1 20.64,20.95 21.59,20 21.59,18.1 23.5,16.19 23.5,14.61 v23.81,14.29 | v33.97,20.95 33.66,20.64 32.98,20.64 IC1.8
IO2
  Bottom 0.406: IC1.29 24.63,32.38 24.13,32.38 20,28.26 20,24.34 R21.2
MCLR
  Top 0.406: ICSP.1 9.38,20.71 R18.1 9.31,19.9 9.84,19.37 11.75,19.37 13.65,21.27 15.88,21.27 16.51,21.91 16.51,26.04 17.6,27.12 IC2.4
MISO  (via drill 0.5)
  Top 0.406: v36.83,23.81 35.88,23.81 35.56,24.13 35.56,26.04 35.88,26.35 35.88,31.75 28.89,38.73 PROG.1
  Bottom 0.406: IC1.2 36.59,23.81 v36.83,23.81
MOSI  (via drill 0.5)
  Top 0.406: v36.51,25.72 36.51,32.07 30.48,38.1 30.48,43.18 29.53,44.13 27.94,44.13 PROG.4
  Bottom 0.406: IC1.1 36.46,25.72 v36.51,25.72
MS1-1  (via drill 0.5)
  Top 0.406: SJ1.1 58.42,4.45 59.69,5.71 v59.69,24.13
  Bottom 0.406: IC1.44 36.46,27.62 37.47,27.62 40.01,25.08 49.85,25.08 50.48,24.45 51.12,24.45 51.75,25.08 52.39,25.08 53.34,24.13 v59.69,24.13
MS1-2
  Bottom 0.406: IC1.11 31.49,18.73 35.56,18.73 39.37,22.54 48.58,22.54 49.21,21.91 65.09,21.91 66.36,23.18 SJ2.1
MS2-1  (via drill 0.5)
  Top 0.406: M1.3 50.8,10.79 v50.8,25.4
  Bottom 0.406: IC1.43 36.27,29.21 36.83,29.21 40.32,25.72 50.48,25.72 v50.8,25.4
MS2-2
  Bottom 0.406: IC1.34 31.49,34.61 35.24,34.61 36.83,33.02 38.73,33.02 42.23,29.53 53.66,29.53 54.61,28.57 60.96,28.57 63.82,25.72 66.99,25.72 69.22,27.94 71.12,27.94 72.39,26.67 72.39,22.54 70.48,20.64 M2.3
MS3-1  (via drill 0.5)
  Top 0.406: M1.4 SJ1.3 58.42,10.16 v58.42,25.08
  Bottom 0.406: IC1.42 35.78,29.84 37.15,29.84 40.64,26.35 52.07,26.35 53.66,24.77 58.1,24.77 v58.42,25.08
MS3-2
  Bottom 0.406: IC1.35 31.99,33.97 34.92,33.97 36.51,32.38 38.42,32.38 41.91,28.89 53.34,28.89 54.29,27.94 60.64,27.94 63.5,25.08 67.31,25.08 69.53,27.3 70.8,27.3 71.75,26.35 71.75,22.86 70.8,21.91 69.53,21.91 68.58,20.95 68.58,19.68 | 68.58,19.68 M2.4 | 68.58,19.68 SJ2.3
MS13-1
  Top 0.406: M1.2 55.24,4.45 SJ1.2
MS13-2
  Top 0.406: M2.2 69.53,23.18 SJ2.2
PWM  (via drill 0.5)
  Top 0.406: v33.66,27.62 33.66,30.8 v29.84,34.61
  Bottom 0.406: IC1.41 33.66,28.85 v33.66,27.62 | v29.84,34.61 28.89,35.56 28.89,36.83 37.2,45.13 Q1.1
PWM-OUT
  Bottom 0.813: Q1.3 39.37,39.5 PWM.3
PWM-RES
  Bottom 0.813: Q1.2 42.18,45.13 R22.2
PWRLED
  Top 0.406: R14.2 61.49,33.55 PWR.A
RA+/SO
  Bottom 0.406: IC1.30 25.12,33.02 23.81,33.02 19.37,28.57 19.37,21.27 20.95,19.68 20.95,17.78 22.86,15.88 22.86,10.79 21.59,9.53 21.59,8.89 20.95,8.26 ST4.6
RA-1A
  Top 1.93: JP1.4 79.38,20.64 80.64,19.37 80.64,16.51 81.6,15.56 M2.12
RA-1B
  Bottom 1.93: JP1.1 M2.11
RA-2A
  Bottom 1.93: JP1.2 79.69,15.56 82.23,18.1 M2.13
RA-2B
  Bottom 1.93: JP1.3 79.06,18.1 81.6,20.64 M2.14
RA-/!SS
  Bottom 0.406: IC1.33 26.61,34.92 22.86,34.92 17.46,29.53 17.46,20.32 19.05,18.73 19.05,12.7 19.68,12.06 ST4.3
RESET  (via drill 0.5)
  Top 0.406: v24.45,27.62 23.07,27.62 C9.2 | v35.56,21.91 35.56,22.23 34.82,22.96 | 34.82,22.96 R20.1 34.08,22.96 34.29,23.18 34.29,23.5 | 34.82,22.96 34.29,23.5 | 34.29,23.5 34.29,26.67 34.61,26.99 34.61,31.11 30.16,35.56 28.89,35.56 26.04,38.42 24.45,38.42 23.81,39.05 PROG.5
  Bottom 0.406: v24.45,27.62 26.35,27.62 27.94,29.21 29.53,29.21 33.02,25.72 33.02,25.12 IC1.4 35.24,22.9 35.24,22.23 v35.56,21.91
RX  (via drill 0.5)
  Top 0.406: v29.21,27.3 29.21,28.57 25.08,32.7 R16.1
  Bottom 0.406: IC1.7 30.48,24.27 30.48,26.35 29.53,27.3 v29.21,27.3
RX(USB)
  Top 0.406: IC2.12 16.72,30.37 18.1,31.75 20,31.75 20.95,32.7 R16.2
SCLK  (via drill 0.5)
  Top 0.406: v36.2,22.86 35.88,22.86 34.92,23.81 34.92,26.35 35.24,26.67 35.24,31.43 30.16,36.51 v29.84,36.51 28.89,36.51 26.35,39.05 PROG.3 | v56.2,31.43 56.62,31.85 R13.1
  Bottom 0.406: IC1.3 36.2,23.08 v36.2,22.86 | v29.84,36.51 30.16,36.51 31.43,35.24 35.56,35.24 37.15,33.66 39.05,33.66 42.55,30.16 54.93,30.16 v56.2,31.43
STATLED
  Top 0.406: R13.2 55.78,33.55 STAT.A
STEP-1  (via drill 0.5)
  Top 0.406: v52.07,24.13 52.07,19.68 M1.7
  Bottom 0.406: IC1.26 25.36,28.26 26.04,28.26 27.62,29.84 29.84,29.84 33.02,26.67 37.47,26.67 39.69,24.45 49.53,24.45 50.16,23.81 51.75,23.81 v52.07,24.13
STEP-2  (via drill 0.5)
  Top 0.406: M2.7 69.22,10.48 63.5,16.19 v63.5,23.18
  Bottom 0.406: IC1.10 31.99,19.37 35.24,19.37 39.05,23.18 48.9,23.18 49.53,22.54 62.87,22.54 v63.5,23.18
SWITCH
  Bottom 3: D1.C 64.88,46.35 60.64,46.35 58.74,44.45 | 58.74,44.45 55.56,41.27 | 55.56,41.27 PWR-SW.COM | 55.56,41.27 PWR-SW.NO 58.74,41.53 58.74,44.45
TX  (via drill 0.5)
  Top 0.406: v28.26,28.26 25.4,31.11 R15.1
  Bottom 0.406: IC1.5 32.38,24.63 32.38,25.4 29.21,28.57 28.57,28.57 v28.26,28.26
TX(USB)
  Top 0.406: IC2.10 20.97,31.02 R15.2
USBLED
  Top 0.406: R19.1 50.06,33.55 USB.A
USBOSC1
  Top 0.406: IC2.2 20.21,25.82 20.64,25.4 20.64,23.5 20.32,23.18 19.43,23.18 X2.P$2 18.8,22.29 17.88,21.38 C8.1
USBOSC2
  Top 0.406: IC2.3 20.52,26.47 21.27,25.72 21.27,23.5 21.59,23.18 22.16,23.18 X2.P$1 23.07,22.26 C7.1
USBSTAT  (via drill 0.5)
  Top 0.406: R19.2 51.02,31.43 v50.48,31.43 | v37.47,34.61 34.92,34.61 31.11,38.42 31.11,43.5 29.84,44.77 27.94,44.77 27.3,45.4 v24.13,45.4 | v16.51,29.53 14.76,27.77 IC2.16
  Bottom 0.406: v50.48,31.43 49.85,30.8 42.86,30.8 39.37,34.29 37.78,34.29 v37.47,34.61 | v24.13,45.4 23.81,45.4 21.91,43.5 21.91,34.92 v16.51,29.53
V+
  Top 1.016: IC3.2 19.93,45.82 C10.1 22.64,45.82 23.5,46.67 29.53,46.67 32.23,43.97 32.23,38.89 33.81,37.31 36.86,37.31 PWM.2
  Top 1.778: PWM.2 37.27,37.02 37.47,36.83 42.86,36.83
  Top 1.93: 44.77,2.54 44.77,1.91 M1.16 38.06,1.91 C4.+
  Top 2.184: C2.+ 82.55,26.04 M2.16 83.19,26.04 83.19,27.94 82.23,28.89 81.28,28.89
  Top 3: PWR-SW.NC 49.59,44.39 47.62,46.35 44.77,46.35 42.86,44.45 42.86,36.83 42.86,35.56 45.4,33.02 45.4,28.89 | 45.4,28.89 45.4,3.17 44.77,2.54 | 45.4,28.89 81.28,28.89 82.55,27.62
VBUS
  Top 0.406: D2.2 4.33,31.31 USB->.1
VIN
  Bottom 3: D1.A 73.23,42.82 J1.CENTRE
VPIC
  Top 0.406: R18.2 10.88,20.77 ICSP.2 10.88,23.41 10.48,23.81 8.57,23.81 8.26,23.5 8.26,22.96 | IC2.1 18.19,25.17 17.14,24.13 17.14,21.59 16.19,20.64 13.97,20.64 12.06,18.73 8.57,18.73 | 8.57,18.73 8.26,19.05 | 8.26,19.05 8.26,22.86 8.26,22.96 | D2.1 2.02,19.25 2.54,18.73 7.94,18.73 | 7.94,18.73 8.26,19.05 | 7.94,18.73 8.57,18.73 | C5.1 8.26,22.96
VUSB
  Top 0.406: IC2.17 10.02,27.12 8.47,28.68 C6.2

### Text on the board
tPlace: =8834 | =882x/498x | 1 2 3 | Jumpers:
tNames: ESTOP | 12V | IO3 / (SPEED)
bNames: Designed By | Thomas Carpenter | (C) 2013-17 | RA | AstroEQ | V4.7-SMD
Reference: This board design is for AstroEQ boards which fit inside the enclosure on an EQ5 Mount. | The board uses some very tricky surface mount components and is not recommended for DIY. | It is a 2 Layer board designed to be sent for manufacture. The AstroEQ-SMD-Gerber.zip file contains the required gerber files. | I use iteadstudio.com 10cm x 5cm prototype service, selecting 1.2mm thick, HASL, 100% electrical check

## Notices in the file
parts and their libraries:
SparkFun: Licensing: CC v3.0 Share-Alike You are welcome to use this library for commercial purposes.
